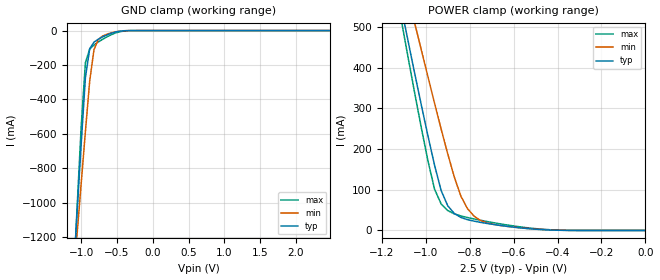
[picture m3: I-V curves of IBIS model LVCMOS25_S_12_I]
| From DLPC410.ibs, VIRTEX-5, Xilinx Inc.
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|   Model LVCMOS25_S_12_I
[Model]  LVCMOS25_S_12_I
Model_type   Input
Polarity   Non-Inverting
Vinl = 0.65
Vinh = 1.85
C_comp   6.0000pF   6.0000pF   6.0000pF
[Model Spec]
Vinl   0.65   0.6   0.7
Vinh   1.85   1.7   2.0
[Temperature Range]   25.0000   85.0000   0.0
[Voltage Range]   2.5000V   2.3000V   2.7000V
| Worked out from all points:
|   GND clamp passes 1 mA (typ) near -0.39 V on its own axis
|   POWER clamp passes 1 mA (typ) near -0.43 V on its own axis
[GND_clamp]
|Voltage   I(typ)   I(min)   I(max)
-2.5V     -11.3A     -8.702A    -13.55A
-1.12V    -1.504A    -1.514A    -1.577A
-1.06V    -1.082A    -1.202A    -1.064A
-1V       -666.6mA   -893.1mA   -565.5mA
-940mV    -273.3mA   -587.1mA   -186.2mA
-880mV    -105.1mA   -292.6mA   -107.5mA
-820mV    -66.91mA   -110.8mA   -83.73mA
-760mV    -50.05mA   -51.73mA   -66.37mA
-700mV    -36.88mA   -31.85mA   -50.72mA
-520mV    -8.293mA   -6.886mA   -14.09mA
-340mV    -253.5uA   -293.6uA   -653.8uA
2.48V     378.6nA    5.297uA    366.7nA
[POWER_clamp]
|Voltage   I(typ)   I(min)   I(max)
-2.49V    4.212A     3.665A     4.661A
-1.11V    543.2mA    639.6mA    512.7mA
-1.08V    463.8mA    573.9mA    423.6mA
-1.05V    384.8mA    508.3mA    336.3mA
-1.02V    307.4mA    442.8mA    251.7mA
-960mV    160.5mA    312.5mA    101.5mA
-930mV    98.04mA    249.2mA    65.3mA
-900mV    60.83mA    188.2mA    48.87mA
-840mV    31.95mA    84.25mA    35.72mA
-780mV    22.84mA    35.01mA    28.28mA
-540mV    4.801mA    5.183mA    6.815mA
0V        384.3nA    408.9nA    427.5nA
